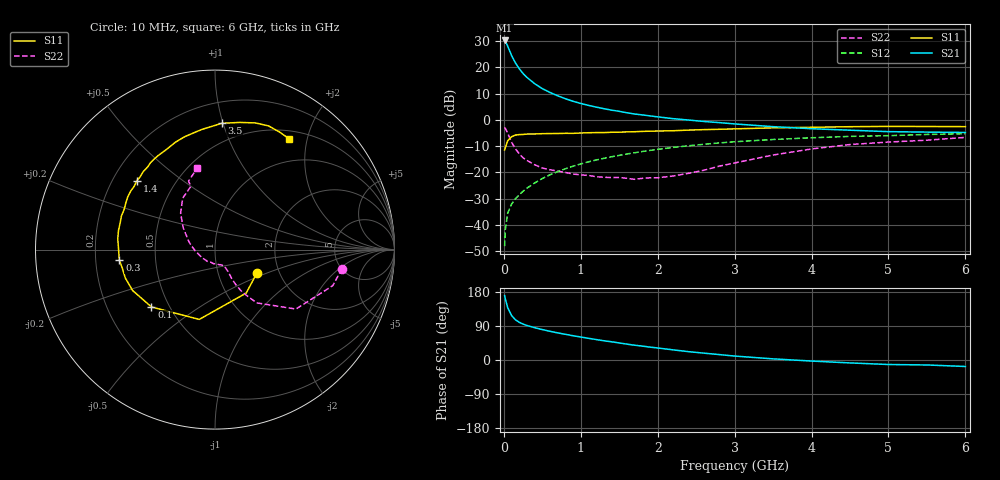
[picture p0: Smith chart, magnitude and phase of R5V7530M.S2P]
! SIEMENS Small Signal Semiconductors
! BFR183
! Si NPN RF Bipolar Junction Transistor in SOT23
! VCE = 0.75 V  IC = 30 mA
! Common Emitter S-Parameters:  May  1996
# GHz  S  MA  R  50
!  f  S11  S21  S12  S22
! GHz  MAG  ANG  MAG  ANG  MAG  ANG  MAG  ANG
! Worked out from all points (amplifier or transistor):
!   36 points, 10 MHz to 6 GHz, reference 50 ohm
!   highest |S21| = 30.3 dB at 10 MHz (marker M1)
!   |S21| within 3 dB of that: start of sweep to 61.89 MHz
!   unconditionally stable (mu >= 1): start of sweep to 19.05 MHz; 176.8 MHz to end of sweep
!   at 250 MHz: K = 1.12, MAG = 20.3 dB, |S12| = -27.2 dB
!   at 1.4 GHz: K = 1.21, MAG = 6.1 dB, |S12| = -14.1 dB
!   at 6 GHz: K = 1.06, MAG = -1.3 dB, |S12| = -5.3 dB
!   S11 on the Smith chart (normalised r, x): 10 MHz: 1.53, -0.44; 100 MHz: 0.40, -0.33; 300 MHz: 0.30, -0.05; 1.4 GHz: 0.30, +0.35; 3.5 GHz: 0.35, +0.99; 6 GHz: 0.61, +1.70
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0.01  0.2673 -29.8  32.7 170.1  0.0039 77.5  0.7158 -8.5
0.02  0.2981 -54.3  31.48 160.7  0.0081 72.5  0.6864 -17.0
0.05  0.3987 -102.7  25.51 138.3  0.0167 63.1  0.5595 -36.3
0.1  0.4769 -137.9  16.95 117.5  0.0246 58.8  0.3765 -52.0
0.15  0.5126 -153.6  12.25 106.3  0.0312 59.7  0.2818 -57.4
0.2  0.524 -162.4  9.451 99.6  0.0372 61.9  0.2248 -59.3
0.25  0.5269 -168.7  7.656 94.7  0.0435 63.3  0.1889 -60.1
0.3  0.536 -173.7  6.463 91.1  0.0498 65.5  0.1687 -59.6
0.4  0.5385 178.5  4.901 85.3  0.0626 67.1  0.1395 -59.5
0.5  0.5452 173.6  3.939 80.2  0.076 68.0  0.1206 -59.8
0.6  0.5482 168.8  3.331 75.7  0.0896 68.4  0.1117 -60.3
0.7  0.5493 163.8  2.879 71.5  0.103 68.0  0.1056 -61.7
0.8  0.5541 160.2  2.532 67.8  0.1166 67.1  0.0993 -64.2
0.9  0.5532 156.4  2.262 64.0  0.1309 66.2  0.0927 -66.8
1.1  0.5681 148.8  1.89 57.3  0.1583 64.2  0.0871 -75.5
1.4  0.5806 138.6  1.534 48.1  0.198 60.2  0.0796 -89.0
1.7  0.5941 129.1  1.293 39.0  0.2358 55.9  0.0735 -108.3
2.2  0.6201 115.8  1.055 26.8  0.2976 48.2  0.085 -146.7
3.5  0.7043 87.0  0.742 3.0  0.4222 27.0  0.2137 145.8
4.5  0.7406 72.4  0.635 -7.7  0.4845 12.6  0.3384 122.1
5.5  0.7472 61.3  0.584 -13.1  0.527 1.5  0.4095 111.1
6  0.7428 56.4  0.575 -17.1  0.5435 -5.7  0.4629 102.5
